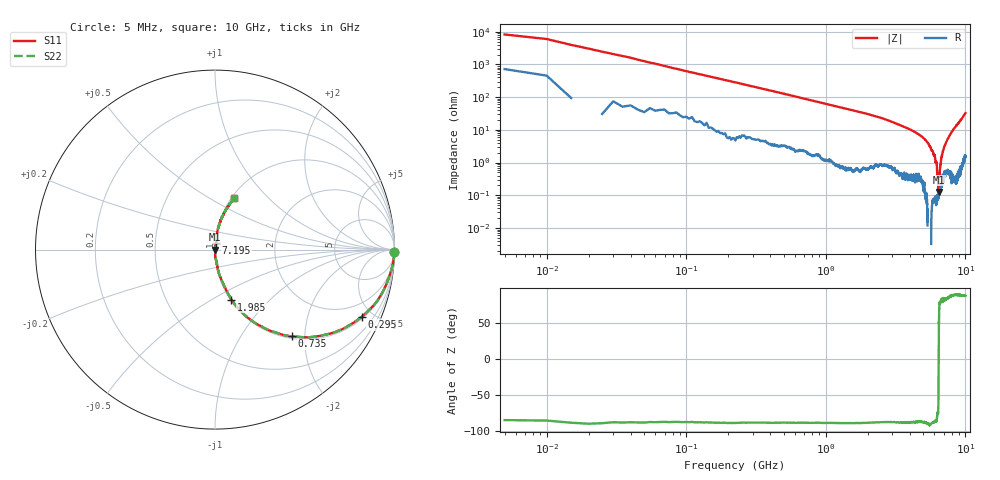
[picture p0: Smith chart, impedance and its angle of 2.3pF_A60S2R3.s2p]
! Amotech Co.,Ltd.
! http://www.amotech.co.kr/
! Part Number: A60S2R3
! These Parameters are Measured in Series Mode Connection
! Operation Temp=25[degC], DC Bias Voltage=0[V]
! Freq. Start=5[MHz] Stop=10[GHz], 2000[Steps]
! Date: Monday, July 13, 2020, 01:26:05
# GHZ S RI R 50.000000
!Freq.(Hz) S11(Real) S11(Imag) S21(Real) S21(Imag) S12(Real) S12(Imag) S22(Real) S22(Imag)
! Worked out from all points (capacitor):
!   2000 points, 5 MHz to 10 GHz, reference 50 ohm
!   read as one part in series: C = 2.55 pF near 55 MHz
!   lowest |Z| = 126 mohm at 6.43 GHz (marker M1)
!   series resonance near 6.441 GHz, so ESL is about 240 pH
!   S11 on the Smith chart (normalised r, x): 5 MHz: open; 295 MHz: 1.11, -4.30; 735 MHz: 1.04, -1.72; 1.985 GHz: 1.01, -0.62; 7.195 GHz: 1.01, +0.07; 10 GHz: 1.03, +0.65
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0.005  0.9988 -0.0121  0.00121 0.0121  0.00121 0.0121  0.9988 -0.0121
0.065  0.9854 -0.1008  0.0146 0.1008  0.0146 0.1008  0.9854 -0.1008
0.105  0.9669 -0.1615  0.0331 0.1615  0.0331 0.1615  0.9669 -0.1615
0.18  0.9218 -0.2575  0.0782 0.2575  0.0782 0.2575  0.9218 -0.2575
0.295  0.8165 -0.3748  0.1835 0.3748  0.1835 0.3748  0.8165 -0.3748
0.735  0.4277 -0.4829  0.5723 0.4829  0.5723 0.4829  0.4277 -0.4829
1.15  0.2337 -0.4148  0.7663 0.4148  0.7663 0.4148  0.2337 -0.4148
1.675  0.1251 -0.3222  0.8749 0.3222  0.8749 0.3222  0.1251 -0.3222
1.985  0.0916 -0.2786  0.9084 0.2786  0.9084 0.2786  0.0916 -0.2786
3.34  0.0244 -0.14  0.9756 0.14  0.9756 0.14  0.0244 -0.14
5.005  0.00462 -0.0558  0.9954 0.0558  0.9954 0.0558  0.00462 -0.0558
5.405  0.0013 -0.0396  0.9987 0.0396  0.9987 0.0396  0.0013 -0.0396
6.03  0.00102 -0.0162  0.999 0.0162  0.999 0.0162  0.00102 -0.0162
6.215  0.000738 -0.00949  0.9993 0.00949  0.9993 0.00949  0.000738 -0.00949
6.43  0.00122 -0.000296  0.9988 0.000296  0.9988 0.000296  0.00122 -0.000296
6.46  0.00137 0.0017  0.9986 -0.0017  0.9986 -0.0017  0.00137 0.0017
6.555  0.00127 0.00549  0.9987 -0.00549  0.9987 -0.00549  0.00127 0.00549
6.67  0.00203 0.0102  0.998 -0.0102  0.998 -0.0102  0.00203 0.0102
6.9  0.00468 0.0218  0.9953 -0.0218  0.9953 -0.0218  0.00468 0.0218
7.195  0.00569 0.0359  0.9943 -0.0359  0.9943 -0.0359  0.00569 0.0359
8.335  0.0151 0.1103  0.9849 -0.1103  0.9849 -0.1103  0.0151 0.1103
10  0.1076 0.2865  0.8924 -0.2865  0.8924 -0.2865  0.1076 0.2865
